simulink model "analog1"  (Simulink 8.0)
settings: Solver=ode3  StartTime=0.0  StopTime=inf  RelTol=1e-3
InitFcn:
  | dt=0.01;
libraries: arduinolib x3

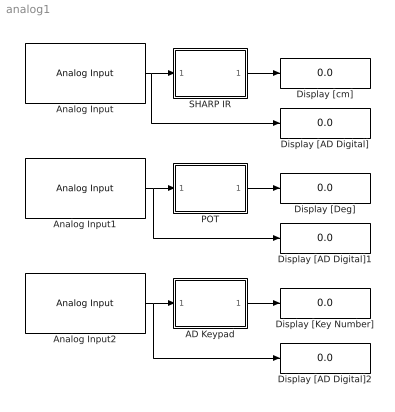
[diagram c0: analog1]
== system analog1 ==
  AD Keypad : MATLAB Function  TreatAsAtomicUnit=on
  Analog Input : arduinolib/Analog Input  pinNumber=0  sampleTime=dt
  Analog Input1 : arduinolib/Analog Input  pinNumber=1  sampleTime=dt
  Analog Input2 : arduinolib/Analog Input  pinNumber=2  sampleTime=dt
  Display [AD Digital] : Display
  Display [AD Digital]1 : Display
  Display [AD Digital]2 : Display
  Display [Deg] : Display
  Display [Key Number] : Display
  Display [cm] : Display
  POT : MATLAB Function  TreatAsAtomicUnit=on
  SHARP IR : MATLAB Function  TreatAsAtomicUnit=on
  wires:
  Analog Input/1 -> Display [AD Digital]/1, SHARP IR/1(u)
  Analog Input1/1 -> Display [AD Digital]1/1, POT/1(u)
  Analog Input2/1 -> Display [AD Digital]2/1, AD Keypad/1(u)
  AD Keypad/1(y) -> Display [Key Number]/1
  SHARP IR/1(y) -> Display [cm]/1
  POT/1(y) -> Display [Deg]/1

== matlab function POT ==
function y = fcn(u)
gain=360/1024;
y=gain*u;

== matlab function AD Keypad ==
function y = fcn(u)
y=-1;
if u>=0 && u<(64-32), y=0; end
if u>=(64-32) && u<(64+32), y=1; end
if u>=(128-32) && u<(128+32), y=2; end
if u>=(192-32) && u<(192+32), y=3; end
if u>=(256-32) && u<(256+32), y=4; end
if u>=(320-32) && u<(320+32), y=5; end
if u>=(384-32) && u<(384+32), y=6; end
if u>=(448-32) && u<(448+32), y=7; end
if u>=(512-32) && u<(512+32), y=8; end
if u>=(576-32) && u<(576+32), y=9; end
if u>=(640-32) && u<(640+32), y=10; end
if u>=(704-32) && u<(704+32), y=11; end
if u>=(768-32) && u<(768+32), y=12; end
if u>=(832-32) && u<(832+32), y=13; end
if u>=(896-32) && u<(896+32), y=14; end
if u>=(960-32) && u<(960+32), y=15; end
if u<0 || u>=(960+32), y=-1; end

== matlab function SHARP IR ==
function y = fcn(u)
gain=5/1024;    % 1024 for 5V %
v=gain*u;

y=0;
if v>=2.9, y=3.5; end
if v>=2.6 && v<2.9, y=4.0; end
if v>=2.2 && v<2.6, y=5.0; end
if v>=1.9 && v<2.2, y=6.0; end
if v>=1.7 && v<1.9, y=7.0; end
if v>=1.5 && v<1.7, y=8.0; end
if v>=1.35 && v<1.5, y=9.0; end
if v>=1.2 && v<1.35, y=10.0; end
if v>=1.0 && v<1.2, y=12.0; end
if v>=0.9 && v<1.0, y=14.0; end
if v>=0.8 && v<0.9, y=16.0; end
if v>=0.7 && v<0.8, y=20.0; end
if v>=0.6 && v<0.7, y=25.0; end
if v>=0.5 && v<0.6, y=30.0; end
if v<0.5, y=40.0; end
